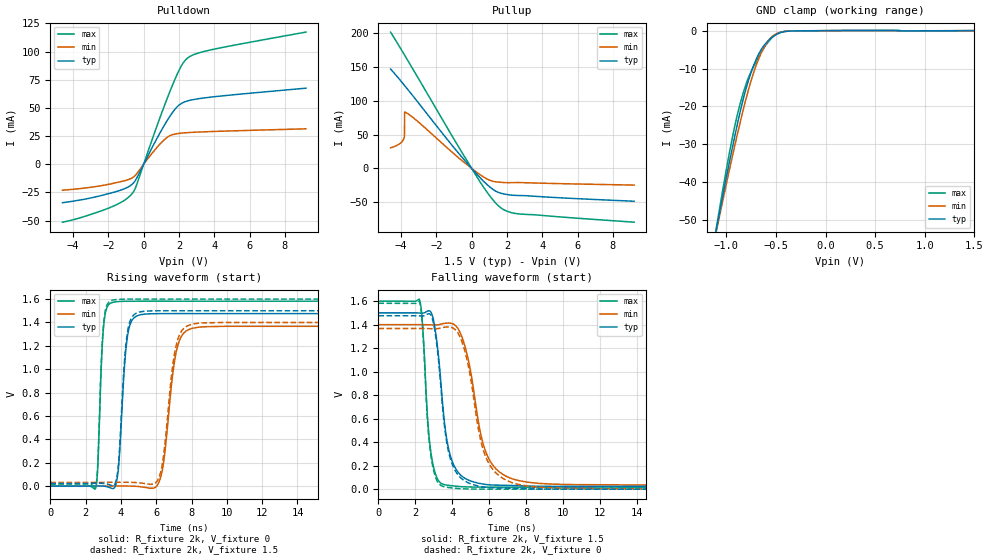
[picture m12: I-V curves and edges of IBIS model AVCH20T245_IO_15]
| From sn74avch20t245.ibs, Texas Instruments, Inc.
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[Model]   AVCH20T245_IO_15
Model_type  I/O
Vinl=0.49
Vinh=1.04
Enable   Active-Low
Vref =   0
Rref =   2000
Cref =   15p
Vmeas =   0.75
| variable   typ   min   max
C_comp   5.30pF   4.64pF   5.87pF
| C_pullup   5.22pF   3.72pF   7.64pF
| C_pulldown   4.91pF   4.33pF   5.57pF
| C_tri-state   5.30pF   4.64pF   5.87pF
[Temperature Range]   40   100   -40
| Ambient temperature   25   85   -40
[Voltage range]   1.5   1.4   1.6
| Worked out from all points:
|   slope of the pulldown table from 0 to 0.225 V, typ, clamps not added: 32.1 ohm
|   slope of the pullup table from 0 to 0.225 V, typ, clamps not added: 33.9 ohm
|   GND clamp passes 1 mA (typ) near -0.50 V on its own axis
|   rising waveform, R_fixture 2k, V_fixture 0: 20-80 % time 361ps typ, 589ps min, 240ps max; typ from 0 V to 1.48 V
|   falling waveform, R_fixture 2k, V_fixture 1.5: 20-80 % time 635ps typ, 1.01ns min, 387ps max; typ from 1.5 V to 0.023 V
|   rising waveform, R_fixture 2k, V_fixture 1.5: 20-80 % time 357ps typ, 576ps min, 239ps max; typ from 0.023 V to 1.5 V
|   falling waveform, R_fixture 2k, V_fixture 0: 20-80 % time 635ps typ, 1.01ns min, 381ps max; typ from 1.48 V to 0 V
[GND Clamp]
| AVCH20T245_IO_15
|   Voltage   I(typ)   I(min)   I(max)
-4.6V     -599.6mA   -548.2mA   -664.6mA
-1.1V     -52.36mA   -52.8mA    -51.85mA
-1.075V   -48.9mA    -49.67mA   -47.95mA
-930mV    -29.68mA   -32.07mA   -27.01mA
-880mV    -23.6mA    -26.34mA   -21.2mA
-830mV    -18.08mA   -20.9mA    -16.41mA
-765mV    -12.13mA   -14.48mA   -11.64mA
-685mV    -6.738mA   -8.147mA   -7.41mA
-605mV    -3.434mA   -3.729mA   -3.946mA
-535mV    -1.679mA   -1.475mA   -1.741mA
-370mV    -121.9uA   -99.54uA   -128.4uA
1.5V      812.2pA    1.554uA    -44.11nA
[Pulldown]
| AVCH20T245_IO_15
|   Voltage   I(typ)   I(min)   I(max)
-4.6V     -34.07mA   -23.01mA   -51.35mA
-1.88V    -25.6mA    -17.43mA   -38.2mA
-1.09V    -21.68mA   -14.59mA   -31.97mA
-625mV    -17.31mA   -11.83mA   -25.44mA
-415mV    -12.94mA   -8.777mA   -18.95mA
595mV     18.22mA    11.97mA    26.91mA
1.265V    37.01mA    23.01mA    55.56mA
1.695V    47.18mA    26.54mA    72.43mA
2.025V    52.71mA    27.44mA    83.88mA
2.495V    56.22mA    28.09mA    94.25mA
3.835V    59.62mA    29.04mA    101.6mA
9.2V      67.51mA    31.46mA    117.2mA
[Pullup]
| AVCH20T245_IO_15
|   Voltage   I(typ)   I(min)   I(max)
-4.6V     146.8mA    30.47mA    201.5mA
-4.1V     131.8mA    36.24mA    180.2mA
-3.85V    123.9mA    43.96mA    169.4mA
-3.81V    122.6mA    49.37mA    167.6mA
-3.805V   122.5mA    83.3mA     167.4mA
-3.785V   121.8mA    83.17mA    166.5mA
-3.155V   101.3mA    71.56mA    138.9mA
175mV     -5.197mA   -3.574mA   -7.497mA
980mV     -26.35mA   -16.94mA   -39.04mA
1.625V    -36.35mA   -20.39mA   -57.65mA
2.595V    -39.89mA   -20.78mA   -66.9mA
9.2V      -48.41mA   -24.54mA   -79.36mA
[Ramp]
| AVCH20T245_IO_15
| variable   typ   min   max
dV/dt_r   0.90/3.76E-10   0.83/5.98E-10   0.96/2.56E-10
dV/dt_f   0.90/6.42E-10   0.83/1.02E-09   0.96/3.95E-10
R_load = 2k
[Rising Waveform]
| AVCH20T245_IO_15
R_fixture =   2k
C_fixture =   0
L_fixture =   0
V_fixture =   0
V_fixture_min = 0
V_fixture_max = 0
|   Time   V(typ)   V(min)   V(max)
0s        19.41nV    97.7nV     527.2pV
2.575ns   904.3uV    -139.8uV   -16.3mV
3.02ns    -186.4uV   133.5uV    1.365V
3.54ns    -21.71mV   690.4uV    1.572V
4.38ns    1.289V     545.3uV    1.581V
5.06ns    1.464V     -4.241mV   1.582V
6.22ns    1.475V     60.26mV    1.582V
7.13ns    1.476V     1.146V     1.582V
8.03ns    1.476V     1.349V     1.582V
40ns      1.476V     1.367V     1.582V
[Falling Waveform]
| AVCH20T245_IO_15
R_fixture =   2k
C_fixture =   0
L_fixture =   0
V_fixture =   1.5
V_fixture_min = 1.4
V_fixture_max = 1.6
|   Time   V(typ)   V(min)   V(max)
0s        1.5V       1.4V       1.6V
2.225ns   1.499V     1.4V       1.612V
2.375ns   1.498V     1.4V       1.429V
2.815ns   1.512V     1.398V     342.5mV
3.15ns    1.272V     1.398V     103.4mV
3.58ns    561.2mV    1.411V     38.01mV
4.6ns     100.8mV    1.259V     20.57mV
5.915ns   38.1mV     277.4mV    17.27mV
7.54ns    29.49mV    74.54mV    17.12mV
40ns      23.4mV     32.34mV    17.1mV
[Rising Waveform]
| AVCH20T245_IO_15
R_fixture =   2k
C_fixture =   0
L_fixture =   0
V_fixture =   1.5
V_fixture_min = 1.4
V_fixture_max = 1.6
|   Time   V(typ)   V(min)   V(max)
0s        23.4mV     32.34mV    17.1mV
2.575ns   24.29mV    32.21mV    1.45mV
3.01ns    23.25mV    32.5mV     1.374V
3.51ns    3.573mV    32.98mV    1.59V
4.37ns    1.315V     32.71mV    1.599V
5.025ns   1.488V     28.47mV    1.6V
6.195ns   1.5V       90.18mV    1.6V
7.1ns     1.5V       1.185V     1.6V
8ns       1.5V       1.383V     1.6V
40ns      1.5V       1.4V       1.6V
[Falling Waveform]
| AVCH20T245_IO_15
R_fixture =   2k
C_fixture =   0
L_fixture =   0
V_fixture =   0
V_fixture_min = 0
V_fixture_max = 0
|   Time   V(typ)   V(min)   V(max)
0s        1.476V     1.367V     1.582V
2.225ns   1.474V     1.367V     1.593V
2.375ns   1.474V     1.367V     1.409V
2.815ns   1.486V     1.365V     316.3mV
3.15ns    1.242V     1.365V     78.77mV
3.565ns   548.6mV    1.378V     20.47mV
4.58ns    79.81mV    1.226V     3.149mV
5.885ns   14.4mV     246.8mV    152.4uV
7.535ns   5.595mV    41.95mV    17.33uV
40ns      225.9nV    540.6nV    168.1nV
